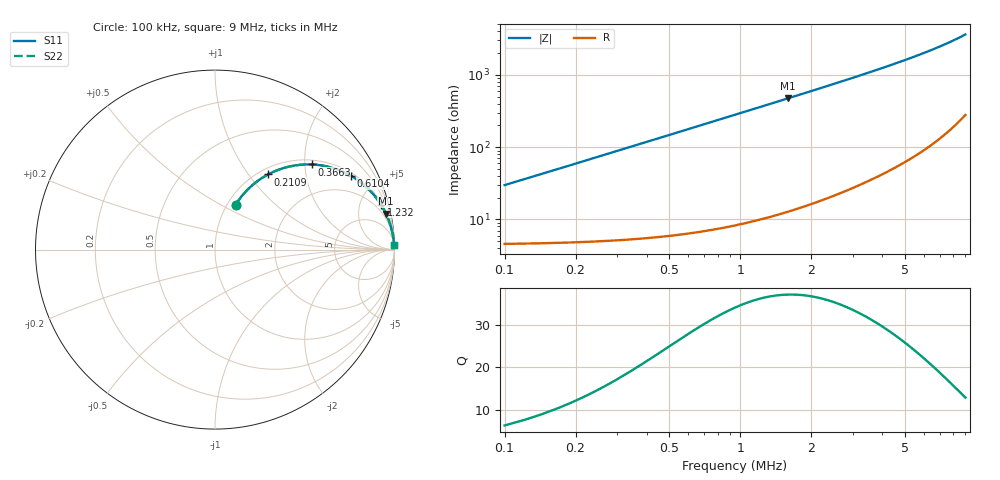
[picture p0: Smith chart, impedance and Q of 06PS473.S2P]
! Coilcraft 0603PS-473 Power Chip Inductor
! 19 February 2003
# MHZ S MA R 50
!Freq  MagS11  AngS11  MagS21  AngS21  MagS12  AngS12  MagS22  AngS22
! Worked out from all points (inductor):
!   403 points, 100 kHz to 9 MHz, reference 50 ohm
!   read as one part in series: L = 47 uH near 144.4 kHz
!   highest Q = 37 at 1.587 MHz (marker M1), where L = 47.4 uH
!   S11 on the Smith chart (normalised r, x): 100 kHz: 1.09, +0.59; 210.9 kHz: 1.10, +1.25; 366.3 kHz: 1.11, +2.16; 610.4 kHz: 1.13, +3.61; 1.232 MHz: 1.20, +7.31; 9 MHz: 7, +72
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0.1  0.275 65.4  0.9202 -15.8  0.9202 -15.8  0.275 65.4
0.14438  0.3795 61.6  0.8847 -22.2  0.8847 -22.2  0.3795 61.6
0.16657  0.4271 59.3  0.8642 -25.2  0.8642 -25.2  0.4271 59.3
0.21095  0.5123 54.8  0.8198 -30.7  0.8198 -30.7  0.5123 54.8
0.27752  0.6163 48.5  0.7504 -38.0  0.7504 -38.0  0.6163 48.5
0.36628  0.7173 41.4  0.6621 -45.8  0.6621 -45.8  0.7173 41.4
0.47723  0.8005 34.5  0.5672 -53.1  0.5672 -53.1  0.8005 34.5
0.5438  0.8351 31.3  0.5192 -56.6  0.5192 -56.6  0.8351 31.3
0.61037  0.8619 28.5  0.4773 -59.5  0.4773 -59.5  0.8619 28.5
0.74351  0.8995 24.1  0.4088 -64.0  0.4088 -64.0  0.8995 24.1
0.87665  0.9239 20.8  0.3558 -67.4  0.3558 -67.4  0.9239 20.8
1.03198  0.9425 17.9  0.3081 -70.4  0.3081 -70.4  0.9425 17.9
1.23169  0.9579 15.2  0.262 -73.2  0.262 -73.2  0.9579 15.2
1.58673  0.973 11.9  0.2059 -76.6  0.2059 -76.6  0.973 11.9
1.89739  0.9803 9.9  0.1728 -78.5  0.1728 -78.5  0.9803 9.9
2.25243  0.9853 8.4  0.1456 -80.0  0.1456 -80.0  0.9853 8.4
3.07346  0.9912 6.1  0.1058 -82.2  0.1058 -82.2  0.9912 6.1
3.76135  0.9936 4.9  0.08525 -83.2  0.08525 -83.2  0.9936 4.9
4.56019  0.9951 3.9  0.0688 -84.0  0.0688 -84.0  0.9951 3.9
6.04692  0.9966 2.8  0.04904 -84.6  0.04904 -84.6  0.9966 2.8
7.53365  0.9972 2.1  0.0364 -84.6  0.0364 -84.6  0.9972 2.1
9  0.9975 1.6  0.02748 -84.0  0.02748 -84.0  0.9975 1.6
